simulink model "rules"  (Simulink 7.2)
settings: Solver=ode45  StartTime=0.0  StopTime=10.0  RelTol=1e-3
undefined symbols (not defined in the file or in its folder): epsilon_K, epsilon_U, OutMax, OutMin
libraries: simulink x2

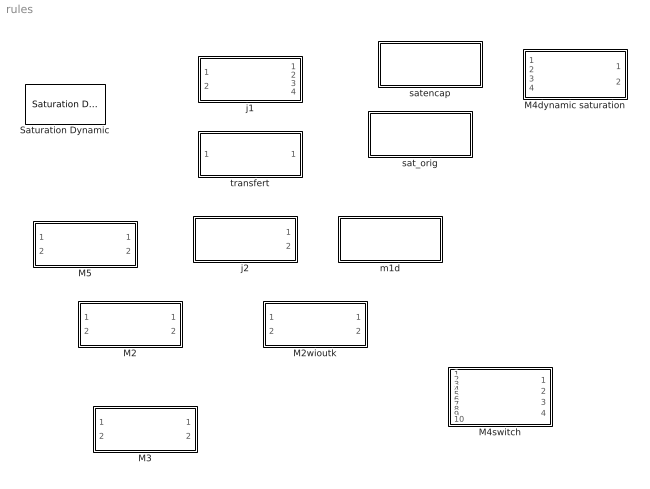
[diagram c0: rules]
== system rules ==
  M2 : Subsystem
  M2wioutk : Subsystem
  M3 : Subsystem
  M4dynamic saturation : Subsystem
  M4switch : Subsystem
  M5 : Subsystem
  Saturation Dynamic : simulink/Discontinuities/Saturation Dynamic  SystemSampleTime=-1  OutMin=[]  OutMax=[]  OutDataTypeStr=Inherit: Same as second input  OutDataType=sfix(16)  OutScaling=2^-10  DoSatur=off
  j1 : Subsystem
  j2 : Subsystem
  m1d : Subsystem
  sat_orig : Subsystem
  satencap : Subsystem
  transfert : Subsystem

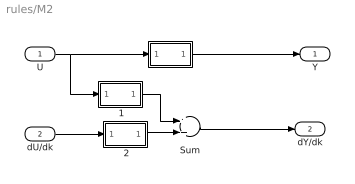
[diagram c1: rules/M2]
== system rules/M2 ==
  U : Inport  OutDataType=sfix(16)  OutScaling=2^0
  dU/dk : Inport  Port=2  OutDataType=sfix(16)  OutScaling=2^0
  " " : Subsystem
  " 1" : Subsystem
  " 2" : Subsystem
  Sum : Sum  OutDataType=sfix(16)  OutScaling=2^0
  Y : Outport  OutDataType=sfix(16)  OutScaling=2^0
  dY/dk : Outport  Port=2  OutDataType=sfix(16)  OutScaling=2^0
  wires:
  U/1 -> " "/1(In1), " 1"/1(In1)
  " "/1(Out1) -> Y/1
  " 1"/1(Out1) -> Sum/1
  dU/dk/1 -> " 2"/1(In1)
  Sum/1 -> dY/dk/1
  " 2"/1(Out1) -> Sum/2

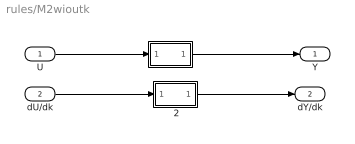
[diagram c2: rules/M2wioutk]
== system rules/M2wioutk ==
  U : Inport  OutDataType=sfix(16)  OutScaling=2^0
  dU/dk : Inport  Port=2  OutDataType=sfix(16)  OutScaling=2^0
  " " : Subsystem
  " 2" : Subsystem
  Y : Outport  OutDataType=sfix(16)  OutScaling=2^0
  dY/dk : Outport  Port=2  OutDataType=sfix(16)  OutScaling=2^0
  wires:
  " 2"/1(Out1) -> dY/dk/1
  dU/dk/1 -> " 2"/1(In1)
  " "/1(Out1) -> Y/1
  U/1 -> " "/1(In1)

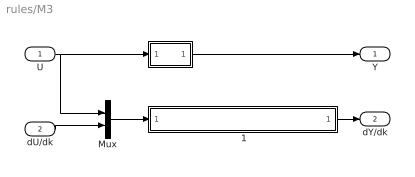
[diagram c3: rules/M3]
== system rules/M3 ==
  U : Inport  OutDataType=sfix(16)  OutScaling=2^0
  dU/dk : Inport  Port=2  OutDataType=sfix(16)  OutScaling=2^0
  " " : Subsystem
  " 1" : Subsystem
  Mux : Mux  Inputs=2
  Y : Outport  OutDataType=sfix(16)  OutScaling=2^0
  dY/dk : Outport  Port=2  OutDataType=sfix(16)  OutScaling=2^0
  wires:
  " "/1(Out1) -> Y/1
  U/1 -> " "/1(In1), Mux/1
  dU/dk/1 -> Mux/2
  Mux/1 -> " 1"/1(In1)
  " 1"/1(Out1) -> dY/dk/1

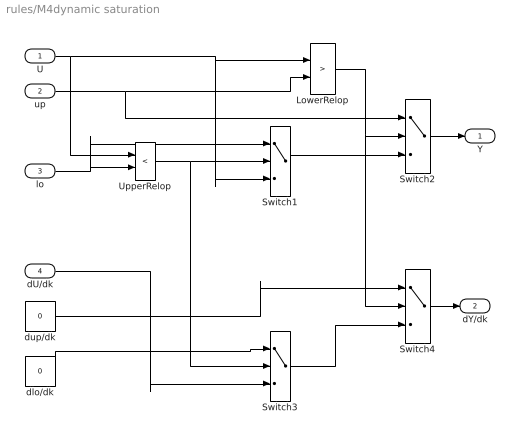
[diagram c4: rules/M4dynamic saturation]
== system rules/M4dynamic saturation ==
  U : Inport  OutDataType=sfix(16)  OutScaling=2^0
  up : Inport  Port=2  OutDataType=sfix(16)  OutScaling=2^0
  lo : Inport  Port=3  OutDataType=sfix(16)  OutScaling=2^0
  dU/dk : Inport  Port=4  OutDataType=sfix(16)  OutScaling=2^0
  LowerRelop : RelationalOperator  DisableCoverage=on  Operator=>  LogicOutDataTypeMode=boolean  OutDataTypeStr=boolean
  Switch1 : Switch  Criteria=u2 ~= 0  OutDataType=sfix(16)  OutScaling=2^0  OutDataTypeStr=Inherit: Inherit via back propagation  ZeroCross=off
  Switch2 : Switch  Criteria=u2 ~= 0  OutMin=OutMin  OutMax=OutMax  OutDataType=OutDataType  OutScaling=OutScaling  OutDataTypeStr=Inherit: Inherit via back propagation  ZeroCross=off
  Switch3 : Switch  Criteria=u2 ~= 0  OutDataType=sfix(16)  OutScaling=2^0  OutDataTypeStr=Inherit: Inherit via back propagation  ZeroCross=off
  Switch4 : Switch  Criteria=u2 ~= 0  OutMin=OutMin  OutMax=OutMax  OutDataType=OutDataType  OutScaling=OutScaling  OutDataTypeStr=Inherit: Inherit via back propagation  ZeroCross=off
  UpperRelop : RelationalOperator  DisableCoverage=on  Operator=<  LogicOutDataTypeMode=boolean  OutDataTypeStr=boolean
  dlo/dk : Constant  Value=0  OutDataType=sfix(16)  OutScaling=2^0
  dup/dk : Constant  Value=0  OutDataType=sfix(16)  OutScaling=2^0
  Y : Outport  OutMin=OutMin  OutMax=OutMax  OutDataType=sfix(16)  OutScaling=2^0
  dY/dk : Outport  Port=2  OutMin=OutMin  OutMax=OutMax  OutDataType=sfix(16)  OutScaling=2^0
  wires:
  up/1 -> Switch2/1, LowerRelop/2
  U/1 -> Switch1/3, LowerRelop/1, UpperRelop/1
  lo/1 -> Switch1/1, UpperRelop/2
  Switch1/1 -> Switch2/3
  Switch2/1 -> Y/1
  LowerRelop/1 -> Switch2/2, Switch4/2
  UpperRelop/1 -> Switch1/2, Switch3/2
  dU/dk/1 -> Switch3/3
  dlo/dk/1 -> Switch3/1
  dup/dk/1 -> Switch4/1
  Switch3/1 -> Switch4/3
  Switch4/1 -> dY/dk/1

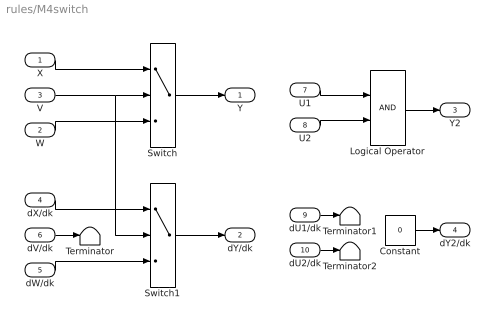
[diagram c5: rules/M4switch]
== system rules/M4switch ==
  X : Inport  OutDataType=sfix(16)  OutScaling=2^0
  W : Inport  Port=2  OutDataType=sfix(16)  OutScaling=2^0
  V : Inport  Port=3  OutDataType=sfix(16)  OutScaling=2^0
  dX/dk : Inport  Port=4  OutDataType=sfix(16)  OutScaling=2^0
  dW/dk : Inport  Port=5  OutDataType=sfix(16)  OutScaling=2^0
  dV/dk : Inport  Port=6  OutDataType=sfix(16)  OutScaling=2^0
  U1 : Inport  Port=7  OutDataType=sfix(16)  OutScaling=2^0
  U2 : Inport  Port=8  OutDataType=sfix(16)  OutScaling=2^0
  dU1/dk : Inport  Port=9  OutDataType=sfix(16)  OutScaling=2^0
  dU2/dk : Inport  Port=10  OutDataType=sfix(16)  OutScaling=2^0
  Constant : Constant  Value=0  OutDataType=sfix(16)  OutScaling=2^0
  Logical Operator : Logic  AllPortsSameDT=off  OutDataTypeMode=boolean  OutDataTypeStr=boolean
  Switch : Switch  Criteria=u2 ~= 0  OutMin=OutMin  OutMax=OutMax  OutDataType=OutDataType  OutScaling=OutScaling  OutDataTypeStr=Inherit: Inherit via back propagation  ZeroCross=off
  Switch1 : Switch  Criteria=u2 ~= 0  OutMin=OutMin  OutMax=OutMax  OutDataType=OutDataType  OutScaling=OutScaling  OutDataTypeStr=Inherit: Inherit via back propagation  ZeroCross=off
  Terminator : Terminator
  Terminator1 : Terminator
  Terminator2 : Terminator
  Y : Outport  OutMin=OutMin  OutMax=OutMax  OutDataType=sfix(16)  OutScaling=2^0
  dY/dk : Outport  Port=2  OutMin=OutMin  OutMax=OutMax  OutDataType=sfix(16)  OutScaling=2^0
  Y2 : Outport  Port=3  OutMin=OutMin  OutMax=OutMax  OutDataType=sfix(16)  OutScaling=2^0
  dY2/dk : Outport  Port=4  OutMin=OutMin  OutMax=OutMax  OutDataType=sfix(16)  OutScaling=2^0
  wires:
  Switch/1 -> Y/1
  X/1 -> Switch/1
  V/1 -> Switch/2, Switch1/2
  W/1 -> Switch/3
  Switch1/1 -> dY/dk/1
  dX/dk/1 -> Switch1/1
  dW/dk/1 -> Switch1/3
  dV/dk/1 -> Terminator/1
  U1/1 -> Logical Operator/1
  U2/1 -> Logical Operator/2
  Logical Operator/1 -> Y2/1
  dU1/dk/1 -> Terminator1/1
  dU2/dk/1 -> Terminator2/1
  Constant/1 -> dY2/dk/1

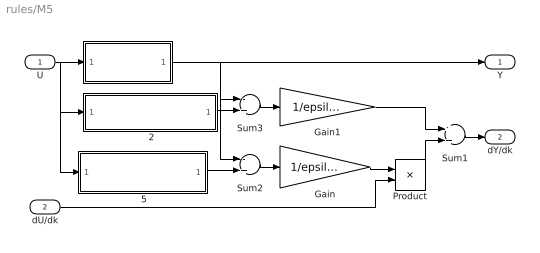
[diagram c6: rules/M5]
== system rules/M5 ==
  U : Inport  OutDataType=sfix(16)  OutScaling=2^0
  dU/dk : Inport  Port=2  OutDataType=sfix(16)  OutScaling=2^0
  " " : Subsystem
  " 2" : Subsystem
  " 5" : Subsystem
  Gain : Gain  Gain=1/epsilon_U  ParameterDataType=sfix(16)  ParameterScaling=2^0  OutDataType=sfix(16)  OutScaling=2^0
  Gain1 : Gain  Gain=1/epsilon_K  ParameterDataType=sfix(16)  ParameterScaling=2^0  OutDataType=sfix(16)  OutScaling=2^0
  Product : Product  OutDataType=sfix(16)  OutScaling=2^0
  Sum1 : Sum  OutDataType=sfix(16)  OutScaling=2^0
  Sum2 : Sum  Inputs=-+  OutDataType=sfix(16)  OutScaling=2^0
  Sum3 : Sum  Inputs=-+  OutDataType=sfix(16)  OutScaling=2^0
  Y : Outport  OutDataType=sfix(16)  OutScaling=2^0
  dY/dk : Outport  Port=2  OutDataType=sfix(16)  OutScaling=2^0
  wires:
  " "/1(Out1) -> Y/1, Sum2/1, Sum3/1
  U/1 -> " "/1(In1), " 5"/1(In1), " 2"/1(In1)
  " 5"/1(Out1) -> Sum2/2
  " 2"/1(Out1) -> Sum3/2
  Sum2/1 -> Gain/1
  dU/dk/1 -> Product/2
  Gain/1 -> Product/1
  Product/1 -> Sum1/2
  Gain1/1 -> Sum1/1
  Sum3/1 -> Gain1/1
  Sum1/1 -> dY/dk/1

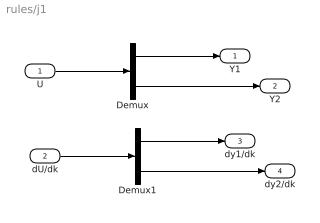
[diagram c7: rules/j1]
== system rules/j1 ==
  U : Inport  OutDataType=sfix(16)  OutScaling=2^0
  dU/dk : Inport  Port=2  OutDataType=sfix(16)  OutScaling=2^0
  Demux : Demux  Outputs=2
  Demux1 : Demux  Outputs=2
  Y1 : Outport  OutDataType=sfix(16)  OutScaling=2^0
  Y2 : Outport  Port=2  OutDataType=sfix(16)  OutScaling=2^0
  dy1/dk : Outport  Port=3  OutDataType=sfix(16)  OutScaling=2^0
  dy2/dk : Outport  Port=4  OutDataType=sfix(16)  OutScaling=2^0
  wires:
  Demux/1 -> Y1/1
  U/1 -> Demux/1
  Demux/2 -> Y2/1
  Demux1/1 -> dy1/dk/1
  dU/dk/1 -> Demux1/1
  Demux1/2 -> dy2/dk/1

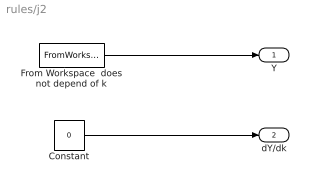
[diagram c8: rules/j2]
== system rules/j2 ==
  Constant : Constant  Value=0  OutDataType=sfix(16)  OutScaling=2^0
  From Workspace  does not depend of k : FromWorkspace  VariableName=simin  SampleTime=0
  Y : Outport  OutDataType=sfix(16)  OutScaling=2^0
  dY/dk : Outport  Port=2  OutDataType=sfix(16)  OutScaling=2^0
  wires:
  From Workspace  does not depend of k/1 -> Y/1
  Constant/1 -> dY/dk/1

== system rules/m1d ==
  note: replaced by
  mixe of original +derivated model here for 2 parameters k1 and k2 : Subsystem
  original model : Subsystem

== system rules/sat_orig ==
  Saturation Dynamic : simulink/Discontinuities/Saturation Dynamic  SystemSampleTime=-1  OutMin=[]  OutMax=[]  OutDataTypeStr=Inherit: Same as second input  OutDataType=sfix(16)  OutScaling=2^-10  DoSatur=off

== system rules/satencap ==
  derivative sturation dynamic block : Subsystem

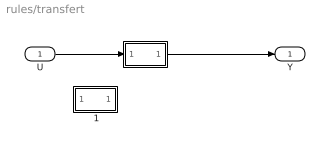
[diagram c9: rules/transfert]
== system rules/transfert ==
  U : Inport  OutDataType=sfix(16)  OutScaling=2^0
  " " : Subsystem
  " 1" : Subsystem
  Y : Outport  OutDataType=sfix(16)  OutScaling=2^0
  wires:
  U/1 -> " "/1(In1)
  " "/1(Out1) -> Y/1

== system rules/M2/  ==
  In1 : Inport  OutDataType=sfix(16)  OutScaling=2^0
  Out1 : Outport  OutDataType=sfix(16)  OutScaling=2^0
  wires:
  In1/1 -> Out1/1

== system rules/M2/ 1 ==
  In1 : Inport  OutDataType=sfix(16)  OutScaling=2^0
  Out1 : Outport  OutDataType=sfix(16)  OutScaling=2^0
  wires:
  In1/1 -> Out1/1

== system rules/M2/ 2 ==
  In1 : Inport  OutDataType=sfix(16)  OutScaling=2^0
  Out1 : Outport  OutDataType=sfix(16)  OutScaling=2^0
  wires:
  In1/1 -> Out1/1

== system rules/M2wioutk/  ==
  In1 : Inport  OutDataType=sfix(16)  OutScaling=2^0
  Out1 : Outport  OutDataType=sfix(16)  OutScaling=2^0
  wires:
  In1/1 -> Out1/1

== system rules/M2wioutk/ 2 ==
  In1 : Inport  OutDataType=sfix(16)  OutScaling=2^0
  Out1 : Outport  OutDataType=sfix(16)  OutScaling=2^0
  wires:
  In1/1 -> Out1/1

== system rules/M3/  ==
  In1 : Inport  OutDataType=sfix(16)  OutScaling=2^0
  Out1 : Outport  OutDataType=sfix(16)  OutScaling=2^0
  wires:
  In1/1 -> Out1/1

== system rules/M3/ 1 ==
  In1 : Inport  OutDataType=sfix(16)  OutScaling=2^0
  Out1 : Outport  OutDataType=sfix(16)  OutScaling=2^0
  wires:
  In1/1 -> Out1/1

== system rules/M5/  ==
  In1 : Inport  OutDataType=sfix(16)  OutScaling=2^0
  Out1 : Outport  OutDataType=sfix(16)  OutScaling=2^0
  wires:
  In1/1 -> Out1/1

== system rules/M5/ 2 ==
  In1 : Inport  OutDataType=sfix(16)  OutScaling=2^0
  Out1 : Outport  OutDataType=sfix(16)  OutScaling=2^0
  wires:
  In1/1 -> Out1/1

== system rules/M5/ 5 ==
  In1 : Inport  OutDataType=sfix(16)  OutScaling=2^0
  Out1 : Outport  OutDataType=sfix(16)  OutScaling=2^0
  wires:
  In1/1 -> Out1/1

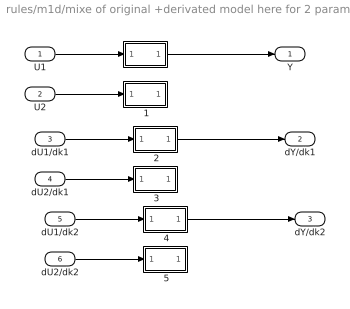
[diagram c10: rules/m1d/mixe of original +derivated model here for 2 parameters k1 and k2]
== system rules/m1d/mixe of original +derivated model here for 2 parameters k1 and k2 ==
  U1 : Inport  OutDataType=sfix(16)  OutScaling=2^0
  U2 : Inport  Port=2  OutDataType=sfix(16)  OutScaling=2^0
  dU1/dk1 : Inport  Port=3  OutDataType=sfix(16)  OutScaling=2^0
  dU2/dk1 : Inport  Port=4  OutDataType=sfix(16)  OutScaling=2^0
  dU1/dk2 : Inport  Port=5  OutDataType=sfix(16)  OutScaling=2^0
  dU2/dk2 : Inport  Port=6  OutDataType=sfix(16)  OutScaling=2^0
  " " : Subsystem
  " 1" : Subsystem
  " 2" : Subsystem
  " 3" : Subsystem
  " 4" : Subsystem
  " 5" : Subsystem
  Y : Outport  OutDataType=sfix(16)  OutScaling=2^0
  dY/dk1 : Outport  Port=2  OutDataType=sfix(16)  OutScaling=2^0
  dY/dk2 : Outport  Port=3  OutDataType=sfix(16)  OutScaling=2^0
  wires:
  U1/1 -> " "/1(In1)
  " "/1(Out1) -> Y/1
  U2/1 -> " 1"/1(In1)
  dU1/dk1/1 -> " 2"/1(In1)
  " 2"/1(Out1) -> dY/dk1/1
  dU2/dk1/1 -> " 3"/1(In1)
  dU1/dk2/1 -> " 4"/1(In1)
  " 4"/1(Out1) -> dY/dk2/1
  dU2/dk2/1 -> " 5"/1(In1)

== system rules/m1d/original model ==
  U1 : Inport  OutDataType=sfix(16)  OutScaling=2^0
  U2 : Inport  Port=2  OutDataType=sfix(16)  OutScaling=2^0
  " " : Subsystem
  Y : Outport  OutDataType=sfix(16)  OutScaling=2^0
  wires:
  " "/1(Out1) -> Y/1
  U1/1 -> " "/1(In1)

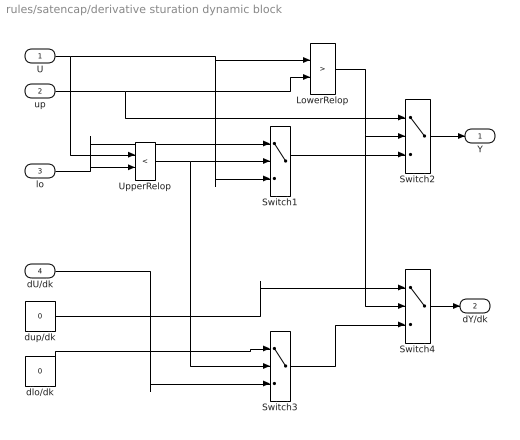
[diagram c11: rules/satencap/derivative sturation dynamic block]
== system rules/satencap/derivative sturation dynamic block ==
  U : Inport  OutDataType=sfix(16)  OutScaling=2^0
  up : Inport  Port=2  OutDataType=sfix(16)  OutScaling=2^0
  lo : Inport  Port=3  OutDataType=sfix(16)  OutScaling=2^0
  dU/dk : Inport  Port=4  OutDataType=sfix(16)  OutScaling=2^0
  LowerRelop : RelationalOperator  DisableCoverage=on  Operator=>  LogicOutDataTypeMode=boolean  OutDataTypeStr=boolean
  Switch1 : Switch  Criteria=u2 ~= 0  OutDataType=sfix(16)  OutScaling=2^0  OutDataTypeStr=Inherit: Inherit via back propagation  ZeroCross=off
  Switch2 : Switch  Criteria=u2 ~= 0  OutMin=OutMin  OutMax=OutMax  OutDataType=OutDataType  OutScaling=OutScaling  OutDataTypeStr=Inherit: Inherit via back propagation  ZeroCross=off
  Switch3 : Switch  Criteria=u2 ~= 0  OutDataType=sfix(16)  OutScaling=2^0  OutDataTypeStr=Inherit: Inherit via back propagation  ZeroCross=off
  Switch4 : Switch  Criteria=u2 ~= 0  OutMin=OutMin  OutMax=OutMax  OutDataType=OutDataType  OutScaling=OutScaling  OutDataTypeStr=Inherit: Inherit via back propagation  ZeroCross=off
  UpperRelop : RelationalOperator  DisableCoverage=on  Operator=<  LogicOutDataTypeMode=boolean  OutDataTypeStr=boolean
  dlo/dk : Constant  Value=0  OutDataType=sfix(16)  OutScaling=2^0
  dup/dk : Constant  Value=0  OutDataType=sfix(16)  OutScaling=2^0
  Y : Outport  OutMin=OutMin  OutMax=OutMax  OutDataType=sfix(16)  OutScaling=2^0
  dY/dk : Outport  Port=2  OutMin=OutMin  OutMax=OutMax  OutDataType=sfix(16)  OutScaling=2^0
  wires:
  Switch4/1 -> dY/dk/1
  Switch3/1 -> Switch4/3
  dup/dk/1 -> Switch4/1
  dlo/dk/1 -> Switch3/1
  dU/dk/1 -> Switch3/3
  UpperRelop/1 -> Switch3/2, Switch1/2
  LowerRelop/1 -> Switch4/2, Switch2/2
  Switch2/1 -> Y/1
  Switch1/1 -> Switch2/3
  lo/1 -> UpperRelop/2, Switch1/1
  U/1 -> UpperRelop/1, LowerRelop/1, Switch1/3
  up/1 -> LowerRelop/2, Switch2/1

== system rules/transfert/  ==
  In1 : Inport  OutDataType=sfix(16)  OutScaling=2^0
  Out1 : Outport  OutDataType=sfix(16)  OutScaling=2^0
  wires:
  In1/1 -> Out1/1

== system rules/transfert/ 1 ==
  In1 : Inport  OutDataType=sfix(16)  OutScaling=2^0
  Out1 : Outport  OutDataType=sfix(16)  OutScaling=2^0
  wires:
  In1/1 -> Out1/1

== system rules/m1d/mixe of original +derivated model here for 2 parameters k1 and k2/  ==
  In1 : Inport  OutDataType=sfix(16)  OutScaling=2^0
  Out1 : Outport  OutDataType=sfix(16)  OutScaling=2^0
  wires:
  In1/1 -> Out1/1

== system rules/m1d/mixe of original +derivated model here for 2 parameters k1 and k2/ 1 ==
  In1 : Inport  OutDataType=sfix(16)  OutScaling=2^0
  Out1 : Outport  OutDataType=sfix(16)  OutScaling=2^0
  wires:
  In1/1 -> Out1/1

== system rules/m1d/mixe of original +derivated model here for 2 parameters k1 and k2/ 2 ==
  In1 : Inport  OutDataType=sfix(16)  OutScaling=2^0
  Out1 : Outport  OutDataType=sfix(16)  OutScaling=2^0
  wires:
  In1/1 -> Out1/1

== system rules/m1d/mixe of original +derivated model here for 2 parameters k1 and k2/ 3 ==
  In1 : Inport  OutDataType=sfix(16)  OutScaling=2^0
  Out1 : Outport  OutDataType=sfix(16)  OutScaling=2^0
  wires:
  In1/1 -> Out1/1

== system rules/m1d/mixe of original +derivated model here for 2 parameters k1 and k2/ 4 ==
  In1 : Inport  OutDataType=sfix(16)  OutScaling=2^0
  Out1 : Outport  OutDataType=sfix(16)  OutScaling=2^0
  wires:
  In1/1 -> Out1/1

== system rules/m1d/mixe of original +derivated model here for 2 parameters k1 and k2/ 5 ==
  In1 : Inport  OutDataType=sfix(16)  OutScaling=2^0
  Out1 : Outport  OutDataType=sfix(16)  OutScaling=2^0
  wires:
  In1/1 -> Out1/1

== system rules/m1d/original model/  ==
  In1 : Inport  OutDataType=sfix(16)  OutScaling=2^0
  Out1 : Outport  OutDataType=sfix(16)  OutScaling=2^0
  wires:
  In1/1 -> Out1/1
